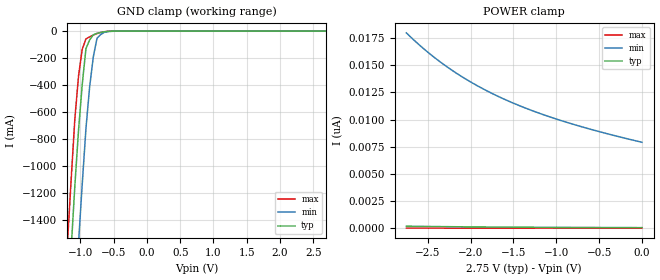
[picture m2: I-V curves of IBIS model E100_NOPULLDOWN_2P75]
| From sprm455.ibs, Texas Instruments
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|   Model Cell E100_NOPULLDOWN_2P75
|IDG09_PE100_NOPULLDOWN_2P75
[Model]   E100_NOPULLDOWN_2P75
Model_type   Input
Polarity   Non-Inverting
Vinl =  0.7V
Vinh =  1.7V
C_comp   1.4352p   1.3677p   1.4356p
[Model Spec]
Vinl   0.7V   0.7V   0.7V
Vinh   1.7V   1.7V   1.7V
[Temperature Range]   25   125   -40
[Voltage Range]   2.75   2.5   3
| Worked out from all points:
|   GND clamp passes 1 mA (typ) near -0.54 V on its own axis
[POWER_clamp]
|   voltage   I(typ)   I(min)   I(max)
-2.75V    182.4pA    17.98nA    2.824pA
-2.667V   173.2pA    17.35nA    2.807pA
-2.5V     157pA      16.2nA     2.602pA
-2.25V    135.9pA    14.71nA    1.954pA
-2V       118.9pA    13.46nA    1.688pA
-1.833V   109.1pA    12.74nA    1.599pA
-1.667V   100.5pA    12.09nA    1.394pA
-1.333V   86.19pA    10.98nA    1.128pA
-916.7mV  72.03pA    9.839nA    1.017pA
-500mV    60.98pA    8.892nA    732.7fA
0V        50.28pA    7.907nA    612.8fA
[GND_clamp]
|   voltage   I(typ)   I(min)   I(max)
-2.75V    -17.11A    -17.95A    -16.64A
-1.194V   -2.105A    -3.008A    -1.577A
-1.139V   -1.621A    -2.516A    -1.105A
-1.083V   -1.151A    -2.031A    -653.7mA
-1.028V   -736.7mA   -1.572A    -333.3mA
-972.2mV  -396.6mA   -1.136A    -134.8mA
-916.7mV  -130.4mA   -725.1mA   -58.05mA
-861.1mV  -65.95mA   -415.2mA   -42.88mA
-805.6mV  -27.97mA   -191.3mA   -29.63mA
-750mV    -16.46mA   -53.29mA   -18.31mA
-638.9mV  -5.249mA   -9.011mA   -4.64mA
2.694V    49.17pA    8.275nA    436.7fA
